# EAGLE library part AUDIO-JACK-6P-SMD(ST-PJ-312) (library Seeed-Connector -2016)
320040007
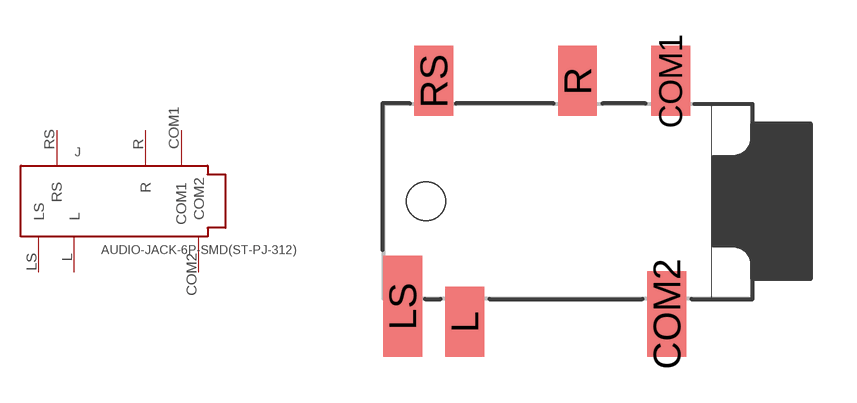
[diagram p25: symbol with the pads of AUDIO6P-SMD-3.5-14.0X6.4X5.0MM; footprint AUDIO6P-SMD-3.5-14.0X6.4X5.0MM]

Designator prefix J

## AUDIO-JACK-6P-SMD(ST-PJ-312) (MPN: ST-PJ-312; VALUE: ST-PJ-312)  [AUDIO6P-SMD-3.5-14.0X6.4X5.0MM]
COM1  COM1
COM2  COM2
L  L
LS  LS
R  R
RS  RS

## Footprint AUDIO6P-SMD-3.5-14.0X6.4X5.0MM (pad centres in mm)
smd 1.27 x 2.286: COM1 -4.572,3.937; L -11.303,-3.937; R -7.62,3.937; RS -12.319,3.937
smd 1.27 x 2.794: COM2 -4.699,-3.683
smd 1.27 x 3.302: LS -13.335,-3.429
hole 1.27 at -12.573,0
